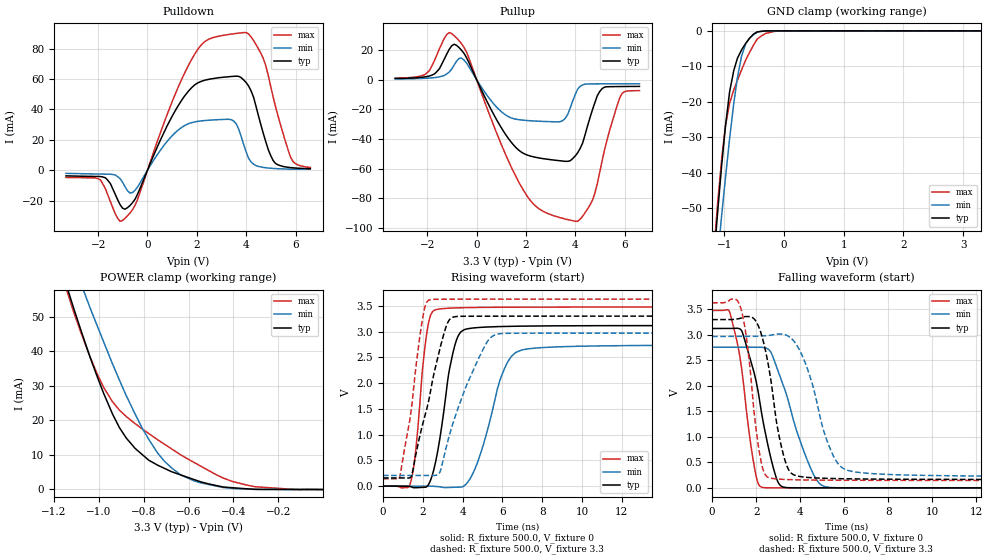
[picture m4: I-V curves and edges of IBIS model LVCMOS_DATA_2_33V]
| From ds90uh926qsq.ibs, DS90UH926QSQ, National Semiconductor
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[Model] LVCMOS_DATA_2_33V
Model_type 3-state
Enable Active-High
Vmeas = 1.65V
Cref = 0.0pF
Rref = 1.0e10
Vref = 0.0V
C_comp   3.52pF   2.88pF   4.05pF
[Voltage Range]   3.3V   2.97V   3.63V
[Temperature Range]   25.0   130.0   -40.0
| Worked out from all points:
|   slope of the pulldown table from 0 to 0.495 V, typ, clamps not added: 26.3 ohm
|   slope of the pullup table from 0 to 0.495 V, typ, clamps not added: 28.9 ohm
|   GND clamp passes 1 mA (typ) near -0.51 V on its own axis
|   POWER clamp passes 1 mA (typ) near -0.47 V on its own axis
|   rising waveform, R_fixture 500.0, V_fixture 0: 20-80 % time 740ps typ, 1.18ns min, 489ps max; typ from 0 V to 3.12 V
|   falling waveform, R_fixture 500.0, V_fixture 0: 20-80 % time 891ps typ, 1.25ns min, 637ps max; typ from 3.13 V to 0 V
|   rising waveform, R_fixture 500.0, V_fixture 3.3: 20-80 % time 1.12ns typ, 1.55ns min, 723ps max; typ from 0.159 V to 3.3 V
|   falling waveform, R_fixture 500.0, V_fixture 3.3: 20-80 % time 723ps typ, 1.1ns min, 533ps max; typ from 3.3 V to 0.162 V
[GND Clamp]
-3.3V     -574.2mA   -508.4mA   -644.1mA
-1.169V   -64.17mA   -75.44mA   -61.85mA
-1.109V   -51.47mA   -64.32mA   -48.84mA
-1.039V   -37.61mA   -51.77mA   -35.92mA
-978.3mV  -27.11mA   -41.75mA   -27mA
-907.9mV  -17.21mA   -30.46mA   -20.42mA
-837.6mV  -11.18mA   -20.45mA   -16.64mA
-706.9mV  -5.349mA   -7.083mA   -10.99mA
-636.5mV  -3.492mA   -3.568mA   -8.136mA
-445.6mV  -275uA     -367.1uA   -2.319mA
-103.9mV  2.878uA    -6.142uA   6.054uA
3.293V    1.011uA    0A         -4.785uA
[POWER Clamp]
-3.3V     572.7mA    510.9mA    640.4mA
-1.139V   58.18mA    70.45mA    57mA
-1.109V   51.99mA    64.99mA    50.92mA
-1.079V   46.04mA    59.55mA    45.39mA
-1.039V   38.33mA    52.66mA    38.41mA
-978.3mV  27.88mA    42.83mA    29.61mA
-907.9mV  17.93mA    31.71mA    23.01mA
-777.3mV  8.489mA    14.52mA    16.22mA
-676.8mV  5.187mA    6.342mA    11.82mA
-576.2mV  2.898mA    2.517mA    7.871mA
-405.4mV  513.4uA    303uA      2.34mA
-3.35mV   -649.4nA   -8.345uA   -32.94uA
[Pullup]
-3.3V     799.7uA    508.2uA    1.021mA
-2.003V   2.146mA    986.4uA    4.683mA
-1.008V   22.85mA    7.191mA    31mA
-606.4mV  19.72mA    14.48mA    24.18mA
891.2mV   -29.36mA   -19.87mA   -39.14mA
1.997V    -50.44mA   -27.47mA   -77.14mA
3.494V    -54.86mA   -27.53mA   -93.42mA
3.997V    -51.41mA   -9.992mA   -95.43mA
4.69V     -20.53mA   -2.872mA   -81.43mA
5.092V    -5.975mA   -2.843mA   -54.22mA
5.896V    -4.624mA   -2.809mA   -9.199mA
6.6V      -4.537mA   -2.797mA   -7.409mA
[Pulldown]
-3.3V     -3.683mA   -2.031mA   -4.727mA
-1.903V   -4.131mA   -2.497mA   -6.36mA
-1.008V   -24.97mA   -7.892mA   -33.01mA
-606.4mV  -21.35mA   -14.67mA   -25.96mA
891.2mV   32.17mA    20.78mA    40.6mA
1.997V    57.1mA     32.07mA    78.51mA
3.394V    61.73mA    33.3mA     89.61mA
3.896V    59.48mA    17.05mA    90.63mA
4.69V     24.49mA    1.897mA    73.76mA
5.092V    6.434mA    1.207mA    48.34mA
5.796V    1.76mA     738.4uA    8.735mA
6.6V      1.071mA    679.9uA    1.86mA
[Rising Waveform]
R_fixture=500.0
V_fixture=0
V_fixture_min=0
V_fixture_max=0
0s        24.71nV    509.5nV    67.81nV
1.4ns     -11.6mV    494.5nV    85.89mV
2.2ns     -12.09mV   1.751uV    2.964V
2.75ns    677.3mV    -8.88mV    3.433V
3.35ns    2.285V     -25.15mV   3.455V
3.9ns     2.99V      -18.87mV   3.463V
4.7ns     3.076V     408.5mV    3.468V
6.2ns     3.101V     2.36V      3.473V
7.25ns    3.107V     2.664V     3.474V
49.98ns   3.12V      2.746V     3.477V
[Falling Waveform]
R_fixture=500.0
V_fixture=0
V_fixture_min=0
V_fixture_max=0
0s        3.126V     2.759V     3.48V
800ps     3.126V     2.759V     3.446V
1.4ns     3.015V     2.759V     2.138V
1.95ns    2.182V     2.76V      332.6mV
2.3ns     1.333V     2.755V     7.354mV
2.65ns    612mV      2.674V     1.107mV
3.1ns     46.87mV    2.164V     650.1uV
4.45ns    647.8uV    407.1mV    291.1uV
5.25ns    422.1uV    13.26mV    206.6uV
49.98ns   6.602uV    16.7uV     3.72uV
[Rising Waveform]
R_fixture=500.0
V_fixture=3.3
V_fixture_min=2.97
V_fixture_max=3.63
0s        159mV      207.3mV    143.3mV
850ps     159mV      207.3mV    183.9mV
1.45ns    215.4mV    207.3mV    1.574V
2ns       1.212V     207.3mV    3.276V
2.4ns     1.864V     207.4mV    3.622V
2.85ns    2.651V     262.9mV    3.628V
3.35ns    3.234V     1.005V     3.629V
4.95ns    3.299V     2.595V     3.63V
5.85ns    3.299V     2.957V     3.63V
49.98ns   3.3V       2.97V      3.63V
[Falling Waveform]
R_fixture=500.0
V_fixture=3.3
V_fixture_min=2.97
V_fixture_max=3.63
0s        3.3V       2.97V      3.63V
1.25ns    3.322V     2.97V      3.59V
1.55ns    3.36V      2.97V      2.965V
2.2ns     3.061V     2.977V     568.2mV
2.75ns    1.852V     3.002V     183.5mV
3.15ns    798.7mV    3.016V     168mV
3.6ns     285mV      2.93V      160mV
5.5ns     182.4mV    630.5mV    149.7mV
6.65ns    174.4mV    302.3mV    147.7mV
49.98ns   162mV      216.6mV    144.5mV
[Ramp]
R_load = 500.0
dV/dt_r   1.872023E0/7.5E-10   1.647456E0/1.2E-9   2.086496E0/5E-10
dV/dt_f   1.882789E0/7.5E-10   1.652056E0/1.1E-9   2.091304E0/5E-10
